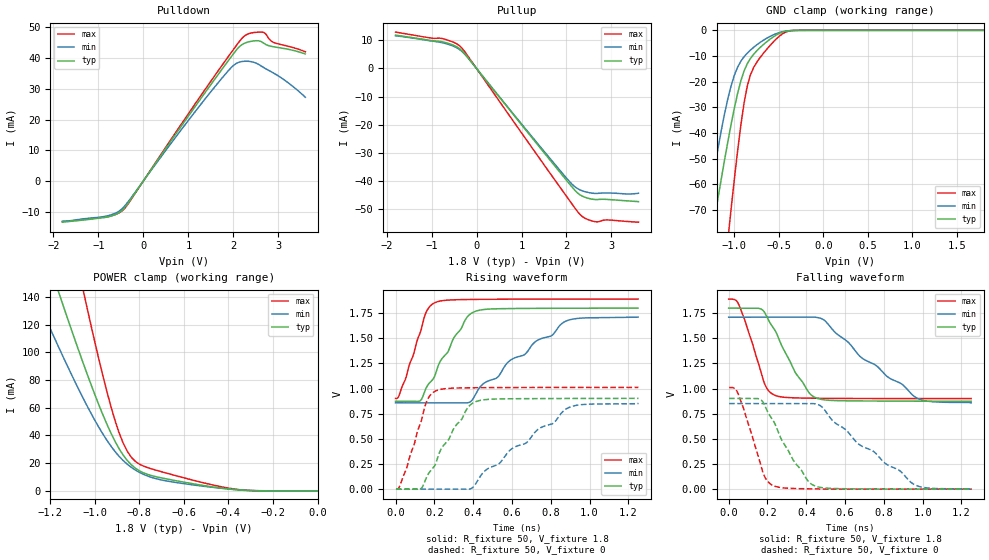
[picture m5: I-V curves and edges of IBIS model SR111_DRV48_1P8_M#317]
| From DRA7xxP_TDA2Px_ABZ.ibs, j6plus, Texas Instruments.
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| Model based on original model for DDR_SEIOPB_H
|   Sub model SR111_DRV48_1P8
[model]   SR111_DRV48_1P8_M#317
|[Description]  [1.8V-I/O-X-X]
|   , ,
|[Input Load]
|[Output Drive]
|Voltage   1.8V
|Mode   I/O
Model_type   I/O
Polarity   Non-Inverting
Enable   Active-Low
Vinl =  0.775
Vinh =  1.025
Cref =  15.0000pF
Rref =  100.0000M
Vref =  0V
Vmeas =  0.9
C_comp   2p   2p   2p
[Model Spec]
Vinl   0.78   0.735   0.825
Vinh   1.02   0.975   1.065
[Receiver Thresholds]
Tslew_ac = 0.5n
Vth = 0.9
Vth_max = 0.945
Vth_min = 0.81
Vinh_ac = 0.2
Vinh_dc = 0.125
Vinl_ac = -0.2
Vinl_dc = -0.125
[Temperature Range]   25   125   -40
[Voltage Range]   1.8   1.71   1.89
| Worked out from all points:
|   slope of the pulldown table from 0 to 0.27 V, typ, clamps not added: 46.9 ohm
|   slope of the pullup table from 0 to 0.27 V, typ, clamps not added: 49.7 ohm
|   GND clamp passes 1 mA (typ) near -0.48 V on its own axis
|   POWER clamp passes 1 mA (typ) near -0.38 V on its own axis
|   rising waveform, R_fixture 50, V_fixture 1.8: 20-80 % time 167ps typ, 371ps min, 93.5ps max; typ from 0.874 V to 1.8 V
|   rising waveform, R_fixture 50, V_fixture 0: 20-80 % time 168ps typ, 372ps min, 93.3ps max; typ from 0 V to 0.903 V
|   falling waveform, R_fixture 50, V_fixture 1.8: 20-80 % time 157ps typ, 342ps min, 94.6ps max; typ from 1.8 V to 0.874 V
|   falling waveform, R_fixture 50, V_fixture 0: 20-80 % time 162ps typ, 354ps min, 94.6ps max; typ from 0.903 V to 0 V
[POWER_clamp]
-1.8V     464.6mA    344.4mA    740.8mA
-1.273V   197mA      143.3mA    314.4mA
-1.164V   144mA      104.2mA    229mA
-1.145V   135.3mA    97.86mA    215mA
-1.055V   93.25mA    67.59mA    146.5mA
-1.036V   85.18mA    61.89mA    133.3mA
-909.1mV  35.72mA    28.41mA    50.73mA
-872.7mV  25.87mA    21.94mA    34.5mA
-818.2mV  16.45mA    15.08mA    21.33mA
-690.9mV  9.084mA    7.592mA    13.42mA
-400mV    1.38mA     1.43mA     2.039mA
0V        227.3nA    761nA      1.176uA
[Pulldown]
-1.8V     -13.45mA   -13.11mA   -13.3mA
-818.2mV  -11.81mA   -11.44mA   -11.72mA
-600mV    -10.83mA   -10.36mA   -10.81mA
-436.4mV  -9.068mA   -8.512mA   -9.288mA
1.255V    26.38mA    24.53mA    27.32mA
1.855V    38.53mA    35.35mA    39.84mA
2.073V    42.76mA    38.34mA    44.25mA
2.291V    45.11mA    39mA       47.65mA
2.618V    45.4mA     37.45mA    48.49mA
2.727V    44.4mA     36.48mA    47.76mA
2.891V    43.71mA    35.16mA    45.15mA
3.6V      41.36mA    27.26mA    42.08mA
[Pullup]
-1.8V     11.9mA     11.66mA    12.97mA
-1.036V   10.04mA    9.888mA    10.91mA
-763.6mV  9.523mA    9.186mA    10.68mA
-490.9mV  8.144mA    7.787mA    9.204mA
-327.3mV  6.377mA    6.133mA    7.311mA
2.018V    -40.23mA   -39.43mA   -46mA
2.182V    -43.37mA   -42.12mA   -49.65mA
2.345V    -45.48mA   -43.6mA    -52.72mA
2.509V    -46.4mA    -44.3mA    -54.07mA
2.673V    -46.74mA   -44.55mA   -54.7mA
2.891V    -46.69mA   -44.38mA   -54.01mA
3.6V      -47.48mA   -44.49mA   -54.81mA
[GND_clamp]
-1.8V     -200.8mA   -187.9mA   -345.9mA
-1.327V   -95.75mA   -76.22mA   -171.1mA
-1.255V   -80.19mA   -60.47mA   -144.9mA
-1.218V   -72.53mA   -52.92mA   -131.9mA
-1.073V   -43.32mA   -26.59mA   -81.54mA
-1.036V   -36.61mA   -21.6mA    -69.55mA
-963.6mV  -24.61mA   -14.37mA   -47.01mA
-854.5mV  -12.98mA   -8.864mA   -21.66mA
-781.8mV  -9.263mA   -6.573mA   -14.36mA
-672.7mV  -5.498mA   -3.827mA   -8.897mA
-345.5mV  -48.81uA   -73.08uA   -79.37uA
1.8V      227.3nA    3.986uA    988nA
[Ramp]
dV/dt_f 0.55627493/0.15687379n 0.51162928/0.34266329n 0.59386695/94.660808p
dV/dt_r 0.54260433/0.16896712n 0.51198135/0.37262907n 0.60761009/93.446947p
R_load = 50
[Rising Waveform]
R_fixture = 50
V_fixture = 1.8
V_fixture_min = 1.71
V_fixture_max = 1.89
0s        873.8mV    858.6mV    901.5mV
50.5ps    873.2mV    858.6mV    1.091V
127.3ps   879.3mV    858.6mV    1.556V
161ps     1.018V     858.6mV    1.772V
206.7ps   1.149V     858.7mV    1.857V
362.8ps   1.694V     857.3mV    1.885V
415.2ps   1.771V     953.1mV    1.887V
587.5ps   1.796V     1.275V     1.889V
876.6ps   1.799V     1.669V     1.89V
1.25ns    1.8V       1.71V      1.89V
[Rising Waveform]
R_fixture = 50
V_fixture = 0
V_fixture_min = 0
V_fixture_max = 0
2.218ps   0V         0V         0V
53.31ps   0V         0V         187.4mV
126.9ps   0V         0V         646.6mV
164.5ps   137mV      0V         889.8mV
212ps     282.9mV    0V         981.1mV
369.6ps   803mV      0V         1.008V
423.9ps   876.9mV    87.06mV    1.009V
593.9ps   898.9mV    394.2mV    1.011V
889.6ps   901.5mV    808.4mV    1.011V
1.252ns   902.5mV    851.6mV    1.011V
[Falling Waveform]
R_fixture = 50
V_fixture = 1.8
V_fixture_min = 1.71
V_fixture_max = 1.89
0s        1.8V       1.71V      1.89V
50.22ps   1.8V       1.71V      1.843V
184.2ps   1.76V      1.71V      1.053V
236.6ps   1.586V     1.71V      935.1mV
344.7ps   1.156V     1.71V      907.6mV
453.1ps   905.4mV    1.709V     904mV
497ps     887.2mV    1.673V     903.2mV
683.5ps   877.2mV    1.31V      901.5mV
968.8ps   874.8mV    907.6mV    900.9mV
1.25ns    873.8mV    858.6mV    900.8mV
[Falling Waveform]
R_fixture = 50
V_fixture = 0
V_fixture_min = 0
V_fixture_max = 0
2.218ps   902.5mV    851.6mV    1.011V
48.51ps   902.7mV    851.6mV    949.5mV
162.3ps   893.2mV    851.6mV    258.4mV
191.1ps   809.8mV    851.6mV    104.7mV
232.1ps   673.2mV    851.6mV    33.61mV
336.4ps   277.7mV    851.4mV    6.53mV
448.6ps   29.28mV    847.7mV    2.399mV
669ps     2.888mV    449.7mV    0V
955.2ps   0V         47.21mV    0V
1.252ns   0V         0V         0V
